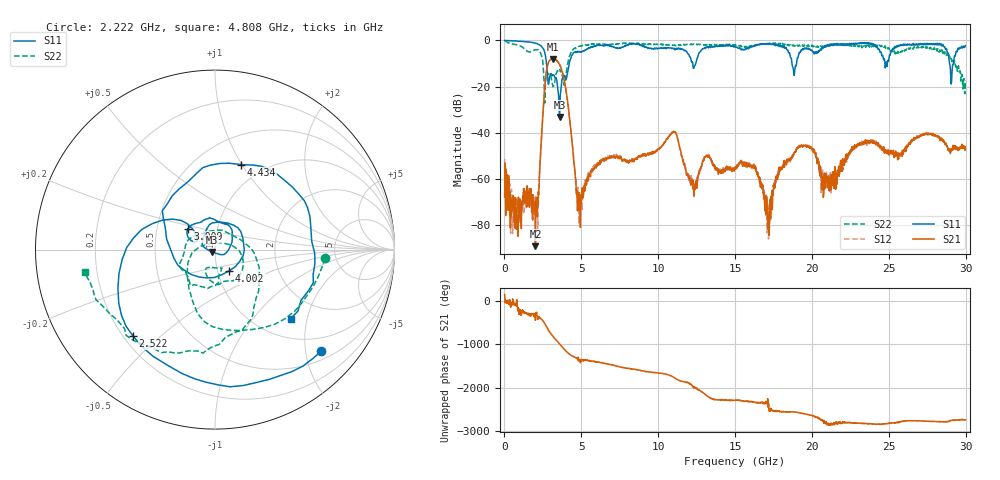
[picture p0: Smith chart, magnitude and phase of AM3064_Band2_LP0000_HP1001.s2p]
# Hz S DB R 50.0
!freq dBS11 angS11 dBS21 angS21 dBS12 angS12 dBS22 angS22
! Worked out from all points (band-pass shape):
!   1600 points, 10 MHz to 29.98 GHz, reference 50 ohm
!   highest |S21| = -7.99 dB at 3.14 GHz (marker M1); lowest = -89.1 dB at 2.016 GHz (marker M2)
!   |S21| within 3 dB of the highest: 2.793 GHz to 3.619 GHz (825.3 MHz wide, 25.7 % of centre)
!   lowest |S11| = -33.2 dB at 3.59 GHz (marker M3), VSWR 1.04, Z = 48.3 - j1.34 ohm
!   |S11| at or under -10 dB: 2.735 GHz to 4.216 GHz (1.481 GHz wide, 42.6 % of centre); 18.7 GHz to 19 GHz (296.4 MHz wide, 1.57 % of centre); 28.95 GHz to 29.2 GHz (255.8 MHz wide, 0.88 % of centre)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
!   |S22| runs from -27.1 to -0.2 dB; largest |S21 - S12| = 0.0096
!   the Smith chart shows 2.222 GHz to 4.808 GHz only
!   S11 on the Smith chart (normalised r, x): 2.222 GHz: 0.68, -2.33; 2.522 GHz: 0.24, -0.41; 3.009 GHz: 0.72, +0.17; 4.002 GHz: 1.14, -0.28; 4.434 GHz: 0.79, +0.99; 4.808 GHz: 1.40, -1.60
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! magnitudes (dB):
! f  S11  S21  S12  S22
! 10 MHz  0.0  -67.8  -51.4  -0.2
! 628.5 MHz  -0.2  -68.1  -79.0  -1.7
! 2.016 GHz  -1.2  -89.1  -69.6  -4.0
! 2.222 GHz  -1.7  -66.9  -64.2  -4.2
! 2.522 GHz  -3.6  -29.7  -29.6  -11.7
! 3.009 GHz  -14.4  -8.3  -8.2  -15.3
! 3.14 GHz  -15.0  -8.0  -7.9  -19.5
! 3.59 GHz  -33.2  -10.5  -10.6  -12.6
! 4.002 GHz  -16.9  -21.6  -21.7  -15.0
! 4.434 GHz  -6.1  -46.4  -46.4  -4.2
! 4.808 GHz  -4.9  -69.7  -67.5  -2.6
! 5.015 GHz  -5.1  -68.1  -71.1  -2.4
! 10 GHz  -3.4  -47.1  -47.0  -1.7
! 11.09 GHz  -3.9  -39.5  -39.6  -2.0
! 12.38 GHz  -11.1  -62.8  -63.4  -1.7
! 15 GHz  -2.5  -55.0  -55.7  -1.8
! 16.32 GHz  -2.2  -54.3  -54.5  -2.1
! 17.16 GHz  -1.7  -81.7  -74.2  -1.5
! 19.99 GHz  -4.3  -46.8  -46.9  -2.1
! 20.82 GHz  -2.8  -57.4  -62.1  -2.3
! 25 GHz  -8.5  -49.1  -48.5  -3.2
! 29.98 GHz  -2.3  -47.3  -47.0  -17.3
